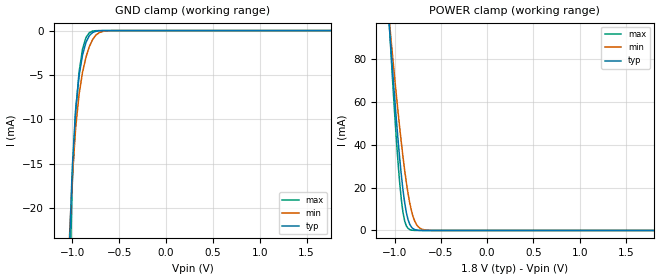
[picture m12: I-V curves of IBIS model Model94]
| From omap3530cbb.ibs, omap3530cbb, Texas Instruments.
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| Model based on original model for IQ0098CS_7LM
|   Sub model IQ0098CS_7LM
[model]   Model94
|[Input Load]
|[Output Drive]
|Voltage   1.8V
|Mode   INPUT
Model_type   Input
Polarity   Non-Inverting
Vinl =  0.63
Vinh =  1.17
C_comp   0.4359588p   0.333509p   0.5556825p
[Model Spec]
Vinl   0.63   0.567   0.6615
Vinh   1.17   1.053   1.2285
[Temperature Range]   25   125   -40
[Voltage Range]   1.8   1.62   1.89
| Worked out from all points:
|   GND clamp passes 1 mA (typ) near -0.84 V on its own axis
|   POWER clamp passes 1 mA (typ) near -0.80 V on its own axis
[POWER_clamp]
-1.8V     607.2mA    493mA      733.8mA
-1.055V   94.58mA    97.12mA    94.87mA
-1.036V   83.61mA    88.55mA    81.27mA
-981.8mV  52.54mA    63.84mA    43.52mA
-945.5mV  34.22mA    48.54mA    22.81mA
-927.3mV  26.14mA    41.36mA    14.7mA
-890.9mV  13.07mA    28.25mA    4.477mA
-836.4mV  2.931mA    12.98mA    432.7uA
-800mV    847uA      6.467mA    76.31uA
-763.6mV  232.1uA    2.845mA    13.67uA
-654.5mV  3.895uA    160.5uA    70.95nA
1.8V      23.69pA    6.013pA    55.72pA
[GND_clamp]
-1.8V     -539.4mA   -380.3mA   -749.6mA
-1.036V   -26.32mA   -24.73mA   -32.34mA
-1V       -15.47mA   -16.64mA   -17.33mA
-963.6mV  -8.866mA   -10.94mA   -9.132mA
-927.3mV  -5.067mA   -7.181mA   -4.683mA
-890.9mV  -2.768mA   -4.717mA   -2.114mA
-854.5mV  -1.349mA   -3.027mA   -800.5uA
-818.2mV  -569.9uA   -1.817mA   -235.6uA
-781.8mV  -214.2uA   -986.5uA   -51.47uA
-745.5mV  -70.13uA   -481.3uA   -9.112uA
-636.4mV  -1.173uA   -35.98uA   -40.16nA
1.764V    20.72pA    95.02pA    35.6pA
